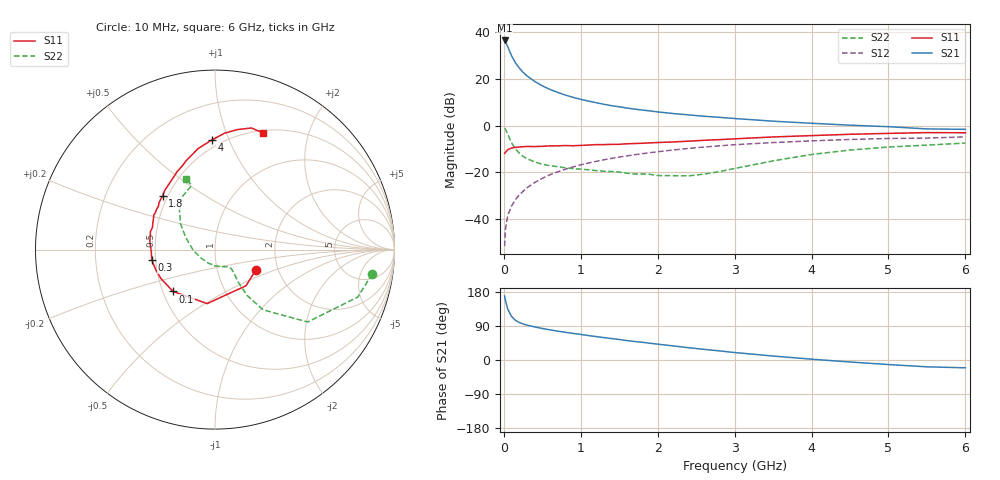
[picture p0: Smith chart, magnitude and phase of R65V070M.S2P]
! SIEMENS Small Signal Semiconductors
! BFR193
! Si NPN RF Bipolar Junction Transistor in SOT23
! VCE = 5 V  IC = 70 mA
! Common Emitter S-Parameters:  May  1996
# GHz  S  MA  R  50
!  f  S11  S21  S12  S22
! GHz  MAG  ANG  MAG  ANG  MAG  ANG  MAG  ANG
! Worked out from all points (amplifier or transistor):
!   36 points, 10 MHz to 6 GHz, reference 50 ohm
!   highest |S21| = 36.5 dB at 10 MHz (marker M1)
!   |S21| within 3 dB of that: start of sweep to 54.69 MHz
!   unconditionally stable (mu >= 1): 346.7 MHz to 2.044 GHz
!   at 250 MHz: K = 0.97, MSG = 25.5 dB, |S12| = -28.2 dB
!   at 1.4 GHz: K = 1.02, MAG = 10.4 dB, |S12| = -14.1 dB
!   at 6 GHz: K = 0.95, MSG = 1.6 dB, |S12| = -4.8 dB
!   S11 on the Smith chart (normalised r, x): 10 MHz: 1.53, -0.37; 100 MHz: 0.57, -0.30; 300 MHz: 0.48, -0.06; 1.8 GHz: 0.47, +0.34; 4 GHz: 0.45, +0.86; 6 GHz: 0.53, +1.35
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0.01  0.2543 -26.5  66.89 168.6  0.0026 79.6  0.8862 -8.8
0.02  0.2654 -49.4  63.81 158.0  0.0058 75.9  0.8384 -18.4
0.05  0.3041 -98.3  49.4 134.7  0.0117 70.2  0.6549 -38.0
0.1  0.33 -135.1  31.48 114.9  0.0188 69.6  0.4294 -51.4
0.15  0.3415 -151.7  22.34 104.8  0.0258 71.7  0.3166 -54.8
0.2  0.3477 -160.2  17.23 99.1  0.0325 73.8  0.2573 -54.9
0.25  0.3529 -167.0  13.9 95.0  0.039 74.2  0.2183 -54.4
0.3  0.3569 -170.9  11.67 92.0  0.0463 75.2  0.1957 -53.0
0.4  0.3554 -178.7  8.856 87.4  0.0601 75.0  0.1664 -51.2
0.5  0.3599 176.9  7.109 83.3  0.0741 75.0  0.1482 -49.9
0.6  0.367 172.2  5.964 79.6  0.0885 74.1  0.1384 -49.8
0.7  0.3682 167.9  5.143 76.1  0.1022 73.3  0.1316 -50.7
0.8  0.3736 164.4  4.51 73.1  0.1161 71.9  0.1245 -51.9
1.1  0.3819 154.2  3.351 64.5  0.1579 68.2  0.1128 -58.4
1.4  0.3962 144.7  2.677 56.6  0.1981 63.8  0.1037 -67.4
1.8  0.4179 134.4  2.156 46.7  0.2501 57.7  0.0919 -86.0
2.2  0.446 125.2  1.815 37.2  0.3001 51.6  0.0845 -114.7
3.5  0.5707 99.5  1.244 10.4  0.4328 31.0  0.1751 157.9
4  0.6101 91.8  1.122 2.2  0.4708 24.0  0.2404 143.2
4.5  0.6509 85.3  1.021 -5.3  0.5041 17.0  0.2989 131.5
5.5  0.7075 73.3  0.849 -18.0  0.5402 3.2  0.381 109.9
6  0.7026 67.7  0.83 -20.6  0.5736 -0.7  0.4224 112.2
